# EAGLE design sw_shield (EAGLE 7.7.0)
CNAME: switch2032; CREVISION: r1; DESIGNER: lamloei
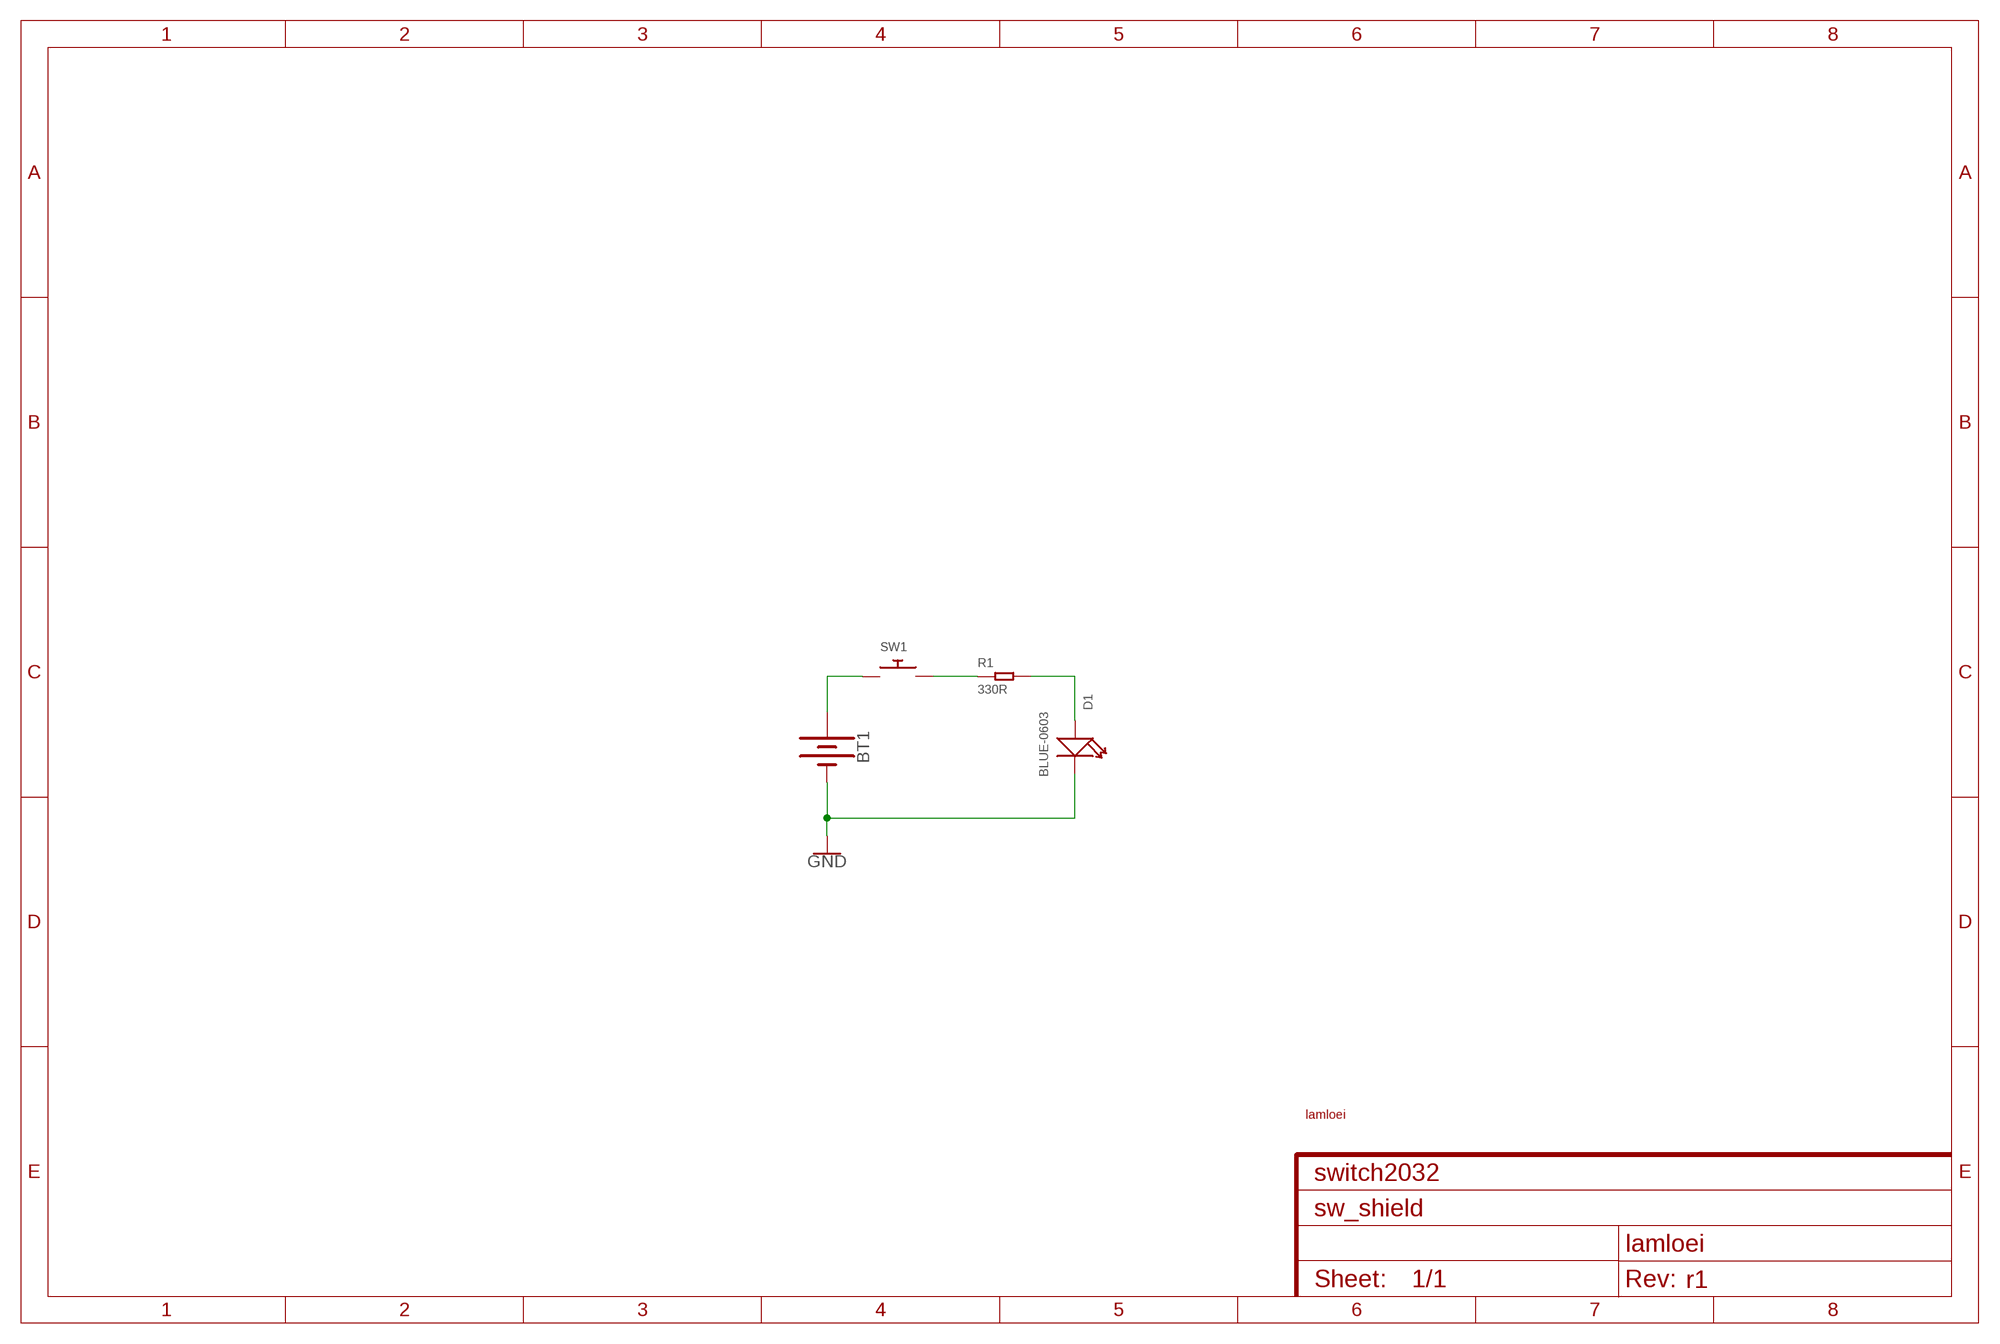
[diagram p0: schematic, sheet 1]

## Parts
BT1  BATTERY-20MM_PTH  [BATTCOM_20MM_PTH]
D1  BLUE-0603  SMD-LED-CLEAR-BLUE(0603)  [LED-0603]
R1  330R  SMD-RES-330R-1%-1/10W(0603)  [R0603]
SW1  SWITCH_PUSHBUTTONEVQ-PE  [TACT_PANA-EVQ]
U$1  LOGO  [LOGO]

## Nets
GND: BT1.2(-) D1.-
N$2: D1.+ R1.2
N$3: R1.1 SW1.P$2
N$4: BT1.1(+) SW1.P$1

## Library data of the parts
BT1 = SparkFun-Batteries:BATTERY: Battery - Single Cell; PROD_ID: BATT-09031; SF_SKU: PRT-00783
D1 = Seeed-LED:SMD-LED-CLEAR-BLUE(0603): 304090045; MPN: 19-217-BHC-ZL1M2RY-3T
R1 = Seeed-Resistor:SMD-RES-330R-1%-1/10W(0603): 301010300; MPN: RC0603FR-07330RL
SW1 = adafruit:SWITCH_PUSHBUTTON: Buttons
U$1 = lib:LOGO

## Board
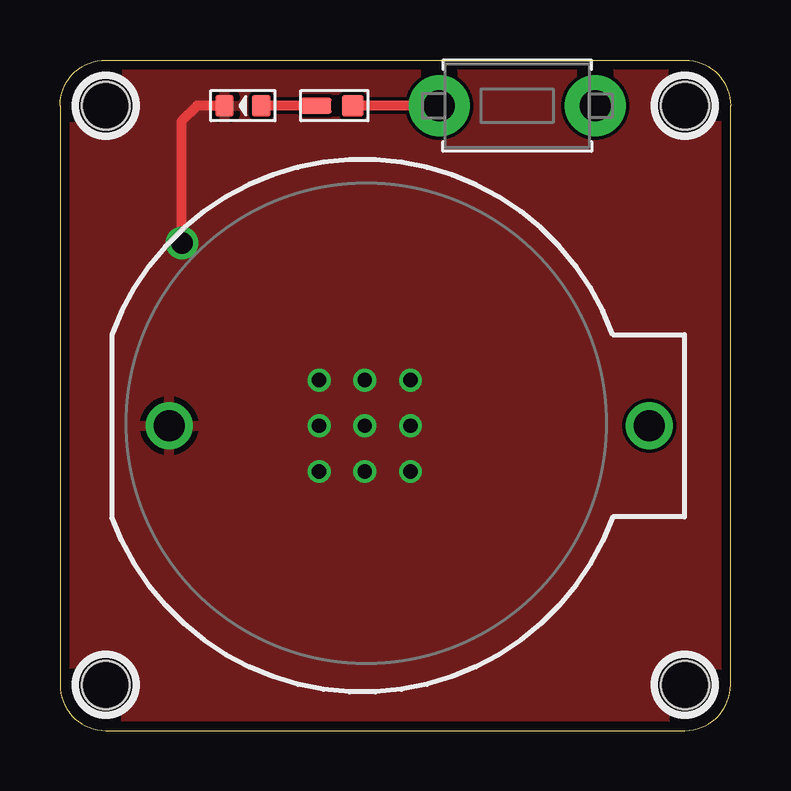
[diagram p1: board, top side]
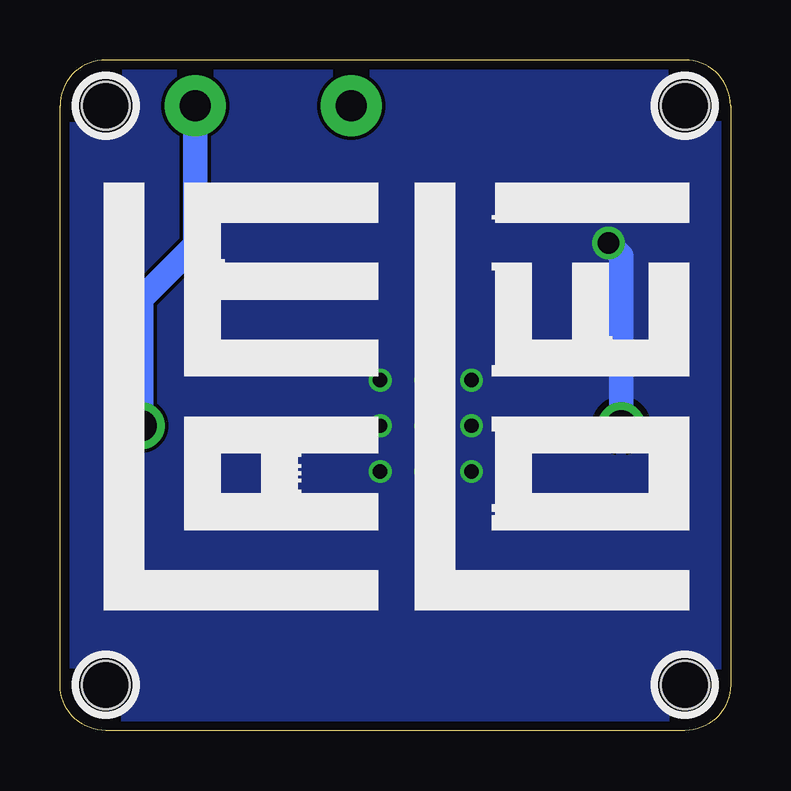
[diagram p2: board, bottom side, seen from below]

Size 27.94 x 27.94 mm. Coordinates in mm from the lower left corner, seen from the top.
Outline: 1.91,0 26.04,0 arc90 27.94,1.91 27.94,26.04 arc90 26.04,27.94 1.91,27.94 arc90 0,26.04 0,1.91 arc90 1.91,0
Copper layers (1*16): Top 0.0356mm / dielectric 1.5011mm / Bottom 0.0356mm
Design rules "oshpark-2layer *": minimum track width 6mil, minimum drill 13mil, track to track 6mil, track to pad 6mil, pad to pad 6mil, via to via 6mil, smd to smd 6mil, copper to edge 15mil, drill to drill 6mil, minimum pad ring 7mil, minimum via ring 7mil, stop-mask expansion 2.5mil, vias tented up to drill 50mil, thermal gap 10mil
Holes 2 mm at 1.91,1.91 26.04,1.91 26.04,26.04 1.91,26.04

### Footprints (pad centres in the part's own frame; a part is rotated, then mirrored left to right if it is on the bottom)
BATTCOM_20MM_PTH = drill 1.3: 1 11.85,0; 2 -8.15,0
LED-0603 = smd 0.762 x 0.889: + -0.762,0; - 0.762,0
R0603 = smd 0.889 x 0.889: 1 0,0.762 | smd 0.66 x 1.27: 2 0,-0.762
TACT_PANA-EVQ = drill 1.3 pad 2.54: P$1 -3.25,0; P$2 3.25,0

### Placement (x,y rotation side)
BT1  12.7,12.7 0 top
D1  7.62,26.04 180 top
R1  11.43,26.04 270 top
SW1  19.05,26.04 180 top
U$1  26.04,5.08 0 bottom

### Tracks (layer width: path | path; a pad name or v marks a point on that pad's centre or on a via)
GND  (via drill 0.6, 0.9)
  Top 0.406: v5.08,20.32 5.08,25.4 5.71,26.04 D1.-
  Bottom 1.016: BT1.2 4.55,19.79 v5.08,20.32
  other vias: 12.7,12.7 12.7,14.61 10.79,14.61 10.79,12.7 14.61,14.61 14.61,12.7 14.61,10.79 12.7,10.79 10.79,10.79
  pour Top: 0,0 27.94,0 27.94,27.94 0,27.94
  pour Bottom: 0,0 27.94,0 27.94,27.94 0,27.94
N$2
  Top 0.406: R1.2 D1.+
N$3
  Top 0.406: SW1.P$2 R1.1
N$4
  Bottom 1.016: BT1.1 24.55,18 22.3,20.25 SW1.P$1

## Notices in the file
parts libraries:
SparkFun-Batteries: Licensing: Creative Commons ShareAlike 4.0 International - https://creativecommons.org/licenses/by-sa/4.0
